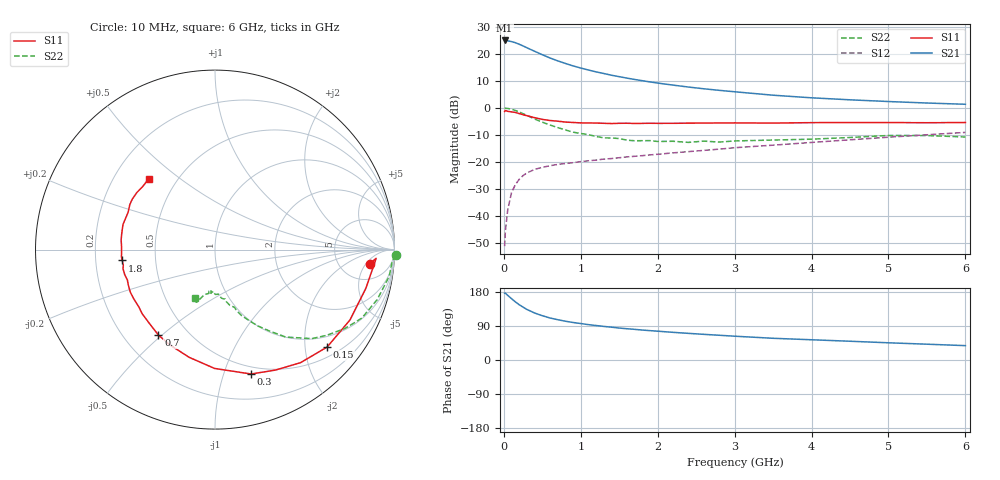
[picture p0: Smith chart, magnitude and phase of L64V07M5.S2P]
!  INFINEON TECHNOLOGIES Small Signal Semiconductors
! BFR380L3 , Si-NPN RF-Transistor in TSLP-3-1
!  Vce=4 V,  Ic=7.5 mA
! Common Emitter S-Parameters:  07. March 2005
#  GHz  S  MA  R  50
! f  S11  S21  S12  S22
! GHz  Mag  Ang  Mag  Ang  Mag  Ang  Mag  Ang
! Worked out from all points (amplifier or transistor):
!   36 points, 10 MHz to 6 GHz, reference 50 ohm
!   highest |S21| = 25.0 dB at 10 MHz (marker M1)
!   |S21| within 3 dB of that: start of sweep to 322.8 MHz
!   unconditionally stable (mu >= 1): 2.38 GHz to 4.675 GHz
!   at 250 MHz: K = 0.20, MSG = 24.0 dB, |S12| = -25.0 dB
!   at 1.4 GHz: K = 0.81, MSG = 15.4 dB, |S12| = -18.7 dB
!   at 6 GHz: K = 0.95, MSG = 5.2 dB, |S12| = -9.0 dB
!   S11 on the Smith chart (normalised r, x): 10 MHz: 10, -6; 150 MHz: 0.72, -2.49; 300 MHz: 0.43, -1.24; 700 MHz: 0.34, -0.49; 1.8 GHz: 0.32, -0.05; 6 GHz: 0.35, +0.39
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0.01  0.8645 -5.2  17.72 176.3  0.0028 83.0  1.01 -1.8
0.02  0.8994 -3.1  17.7 176.4  0.0053 87.4  0.9896 -3.6
0.05  0.868 -14.3  17.46 170.6  0.013 83.7  0.982 -8.7
0.1  0.8482 -27.5  16.87 161.9  0.0274 77.0  0.9459 -17.1
0.15  0.8276 -41.0  16.1 153.4  0.0384 70.1  0.9029 -25.0
0.2  0.7899 -52.9  15.08 145.8  0.0482 64.9  0.8474 -31.2
0.25  0.7511 -63.3  14.04 139.5  0.0565 60.1  0.7845 -37.5
0.3  0.7219 -73.8  12.98 133.4  0.0632 56.9  0.7327 -42.6
0.4  0.6621 -90.2  11.19 124.0  0.0734 51.3  0.6271 -51.0
0.5  0.6174 -103.4  9.655 116.9  0.0802 48.1  0.5472 -56.1
0.6  0.5882 -114.9  8.404 110.9  0.0858 46.3  0.4857 -60.9
0.7  0.571 -123.5  7.443 106.4  0.0907 45.5  0.4351 -64.6
0.9  0.5406 -138.7  6.004 99.0  0.0977 45.0  0.3579 -70.6
1.1  0.5293 -148.8  5.035 93.3  0.1059 46.0  0.322 -75.0
1.4  0.5167 -160.8  4.035 86.6  0.1165 47.8  0.2797 -79.8
1.8  0.5204 -173.3  3.2 79.0  0.1318 50.8  0.2491 -86.4
2.2  0.5212 178.0  2.65 73.0  0.1483 53.1  0.243 -90.9
2.8  0.5296 166.8  2.122 65.3  0.1739 56.5  0.2347 -98.5
3.5  0.5268 156.7  1.725 57.3  0.2059 57.9  0.2561 -102.6
4.5  0.5396 148.7  1.418 49.5  0.2588 60.2  0.2853 -106.7
5.5  0.5346 139.1  1.237 41.7  0.3202 59.4  0.3102 -110.5
6  0.5399 133.1  1.173 37.9  0.3543 58.2  0.2914 -112.2
